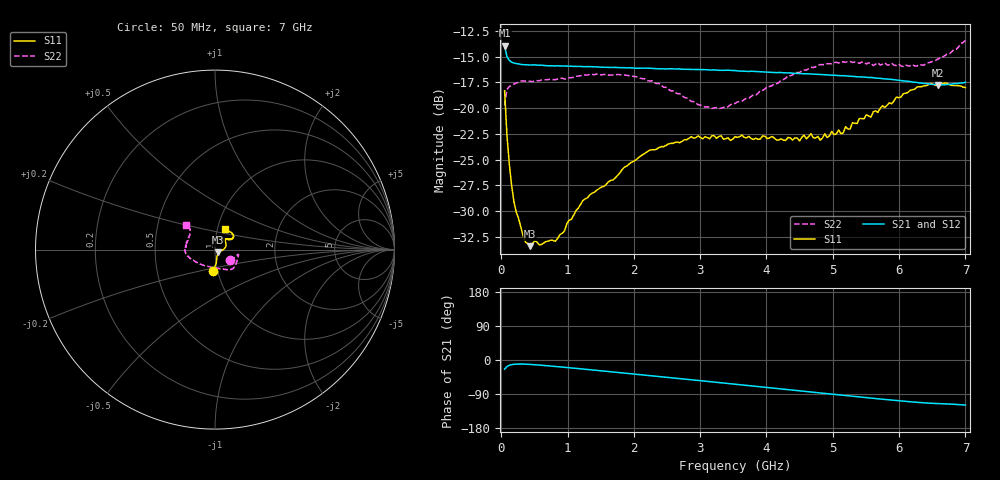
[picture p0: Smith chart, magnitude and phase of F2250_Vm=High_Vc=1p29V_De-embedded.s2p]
! Integrated Device Technology
! Corporate Headquarters
! 6024 Silver Creek Valley Road
! San Jose, CA 95138  USA
! Phone:  1-408-284-8200
! Toll Free:  1-800-223-1366
! Webpage:  http://www.idt.com/
! Timing and RF Division
! 515 Groton Road, Suite 102
! Westford, MA 01886-6024
! Device:  F2250
! Description: Voltage Variable RF Attenuator
! Frequency:  50.0 -  6000.00 MHz
! Package:  3x3 mm Thin QFN Plastic Package: 16 pin
! Ports:  2 RF, 3 DC
!  Pin  1  = GND
!  Pin  2  = NC
!  Pin  3  = RF1  = Port 1
!  Pin  4  = NC
!  Pin  5  = GND
!  Pin  6  = GND
!  Pin  7  = GND
!  Pin  8  = GND
!  Pin  9  = NC
!  Pin 10  = RF2  = Port 2
!  Pin 11  = NC
!  Pin 12  = GND
!  Pin 13  = GND
!  Pin 14  = VCNTRL
!  Pin 15  = VDD
!  Pin 16  = VMODE
! Vcntrl:  1.290 Volts
! Vmode:  +3.300 Volts
! Vdd:  +3.30  Volts
! Current:  1.331 mA
! Data:  The device was measured on a the F2250 evaluation board which has
!  individual transmission lines to the RF pins.  Data was collected
!  using a calibrated network analyzer.  The evaluation board was
!  de-embedded using a TRL calibration technique.
!  The reference plane is the edge of the package pin.
! Misc:  SN 10
!  Action Tracker AT0258
! Date Measured:  2014-11-26
! Date:  2015-10-15  MJV
! Note:
!  Integrated Device Technology supplies this data as a sample of measured
!  data at the package pin for this product.  Your particular data for this
!  product may vary.
!  Data was taken at 25 degrees C.
!  Integrated Device Technology reserves the right to change this data at anytime.
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# GHz S dB R 50
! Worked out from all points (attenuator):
!   201 points, 50 MHz to 7 GHz, reference 50 ohm
!   highest |S21| = -13.93 dB at 50 MHz (marker M1); lowest = -17.8 dB at 6.583 GHz (marker M2)
!   lowest |S11| = -33.4 dB at 432.2 MHz (marker M3), VSWR 1.04, Z = 51.6 - j1.46 ohm
!   |S11| at or under -10 dB: start of sweep to end of sweep
!   |S22| runs from -20.0 to -13.4 dB; largest |S21 - S12| = 0.00058
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0.05  -18.32 -94.6  -13.93 -24.0  -13.92 -24.0  -19.74 -35.5
0.08475  -22.56 -84.4  -15.00 -17.4  -14.99 -17.4  -18.19 -17.8
0.1195  -25.37 -80.1  -15.37 -14.1  -15.36 -14.0  -17.91 -13.1
0.189  -29.03 -69.9  -15.63 -11.4  -15.61 -11.4  -17.67 -11.8
0.328  -32.39 -46.8  -15.79 -10.8  -15.77 -10.8  -17.36 -13.0
0.43225  -33.40 -41.6  -15.83 -11.6  -15.81 -11.6  -17.39 -14.7
0.50175  -32.89 -33.0  -15.81 -12.5  -15.83 -12.5  -17.38 -17.3
0.8145  -32.93 -17.6  -15.91 -17.0  -15.91 -17.0  -17.24 -26.1
1.2315  -28.97 -11.1  -15.98 -23.8  -15.99 -23.8  -16.78 -36.6
1.857  -25.74 4.9  -16.08 -34.4  -16.09 -34.5  -16.79 -48.4
2.37825  -23.83 19.0  -16.19 -43.5  -16.16 -43.5  -17.61 -59.3
3.07325  -22.77 40.9  -16.27 -55.8  -16.26 -55.9  -19.90 -89.7
3.525  -22.77 55.7  -16.36 -64.0  -16.39 -64.0  -19.55 -120.0
4.7065  -22.89 65.0  -16.71 -85.1  -16.69 -85.1  -16.07 -167.0
5.15825  -22.40 47.4  -16.86 -93.2  -16.85 -93.2  -15.51 -176.5
5.193  -21.80 47.8  -16.87 -93.8  -16.87 -93.8  -15.56 -177.3
5.2625  -22.02 44.2  -16.91 -95.0  -16.90 -95.0  -15.47 -178.3
5.29725  -21.42 43.6  -16.93 -95.6  -16.91 -95.7  -15.57 -179.3
5.85325  -19.49 33.5  -17.20 -105.2  -17.19 -105.4  -15.81 166.6
6.27025  -17.97 34.4  -17.52 -111.7  -17.52 -111.7  -15.92 153.4
6.583  -17.72 41.3  -17.76 -115.0  -17.74 -115.1  -15.25 143.2
7  -18.01 63.0  -17.50 -118.9  -17.51 -119.0  -13.44 139.3
